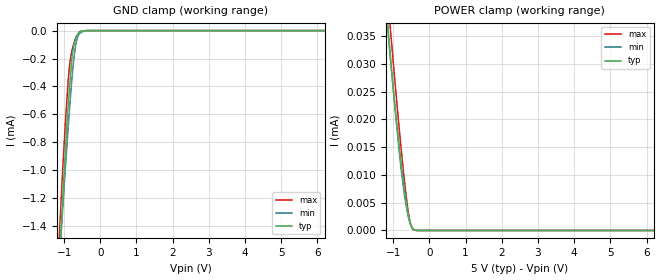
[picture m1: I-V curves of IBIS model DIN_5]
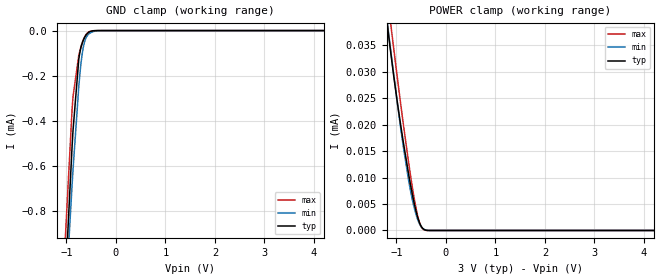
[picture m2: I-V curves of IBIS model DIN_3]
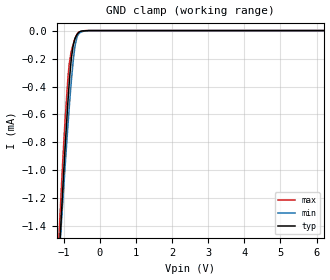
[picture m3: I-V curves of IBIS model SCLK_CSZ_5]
| Texas Instruments Incorporated
| 256 Taps, Dual Channel Digital Potentiometer with SPI Interface and Non-Volatile Memory
| Marketing part#   Voltage Range   Package-type   #pins/pkg drawing
| TPL0202-10MRTE   2.7V - 5.5V   QFN / RTE   16-pin RTE
| TPL0202-10MRUC   2.7V - 5.5V   QFN / RTE   14-pin RUC
[IBIS Ver]   4.1
[File name]   tpl0202.ibs
[File Rev]   1.0
[Date]   01/26/2012
[Source]   Model built from TISPICED simulations at:
   Texas Instruments Incorporated.
   Analog-eLab, HPA
   12500 TI Blvd
   Dallas, TX -75243
   For Support e-mail: elab_ibis@list.ti.com
[Notes]   Revision History
   Rev 1.0: 01/26/2012
   - ccomp values are based on PVT settings:
   WEAK: Low Voltage, High Temperature, Weak Process
   NOM: Nominal Voltage, Nominal Temperature, Nominal Process
   STRONG: High Voltage, Low Temperature, Fast Process
   - User may change ccomp in the order of number values as
   per end simulator used
   - C_comp although listed in numberical order of value are obtained from varying PVT conditions.
   For PVT conditions for eachspecific value, refer to the buffer description under repective [Model].
   IBIS model user is responsible for using appropriate C_comp to simulate for Signal Integrity.
   GND Clamps for DIN adn SCLK_CSZ models are non-monotonic and reflect actual circuit behavior
[Disclaimer] This model is designed as an aid for customers of Texas Instruments.
 TI and its licensors and suppliers make no warranties, either expressed
 or implied, with respect to this  model, including the warranties of
 merchantability or fitness for a particular purpose.
 The model is provided solely on an "as is" basis. The entire risk as to
 its quality and performance is with the customer.
[Copyright] (C)Copyright 2012 Texas Instruments Incorporated.
   All rights reserved.
|   Component TPL0202RTE
[Component]   TPL0202RTE
[Manufacturer]  Texas Instruments Incorporated
[Package]   |16-pin QFN RTE package
|   typ   min   max
R_pkg   0.05510   0.00044   0.09181
L_pkg   0.95615nH   0.09191nH   1.65005nH
C_pkg   0.16177pF   0.10625pF   0.22785pF
[Pin] signal_name   model_name   R_pin   L_pin   C_pin
 1   VDD   POWER   0.05907   1.02864n   0.16975p
 2   SCLK   SCLK_CSZ   0.05510   0.95615n   0.18540p
 3   DIN   DIN   0.05093   0.88345n   0.17719p
 4   CSB   SCLK_CSZ   0.05513   0.95780n   0.16776p
 5   NC   NC   0.00044   0.09191n   0.10625p
 6   NC   NC   0.00047   0.09439n   0.12678p
 7   GND   GND   0.06684   1.17207n   0.19414p
 8   NC   NC   0.00045   0.09475n   0.11241p
 9   NC   NC   0.00044   0.09191n   0.10625p
10   LB   NC   0.07541   1.33519n   0.21758p
11   WB   NC   0.08043   1.43607n   0.22785p
12   HB   NC   0.09181   1.65995n   0.21502p
13   LA   NC   0.05634   0.97306n   0.16177p
14   WA   NC   0.05052   0.87083n   0.17710p
15   HA   NC   0.05460   0.94813n   0.18216p
16   WB   NC   0.00045   0.09475n   0.11241p
|   Component TPL0202RUC
[Component]   TPL0202RUC
[Manufacturer]  Texas Instruments Incorporated
[Package]   |14-pin QFN RUC package
|   typ   min   max
R_pkg   0.03933   0.00040   0.04871
L_pkg   0.52208nH   0.16184nH   0.65360nH
C_pkg   0.12170pF   0.10389pF   0.14505pF
[Pin] signal_name   model_name   R_pin   L_pin   C_pin
 1   VDD   POWER   0.04871   0.65360n   0.11213p
 2   SCLK   SCLK_CSZ   0.03996   0.53951n   0.12170p
 3   DIN   DIN   0.04778   0.62664n   0.14505p
 4   CSB   SCLK_CSZ   0.04046   0.53776n   0.13936p
 5   GND   GND   0.04342   0.57381n   0.14139p
 6   LB   NC   0.04543   0.60528n   0.12661p
 7   WB   NC   0.03966   0.54784n   0.10459p
 8   HB   NC   0.03951   0.54862n   0.10389p
 9   NC   NC   0.00040   0.16960n   0.09156p
10   NC   NC   0.00040   0.16268n   0.10790p
11   NC   NC   0.00040   0.16184n   0.10796p
12   LA   NC   0.03864   0.52208n   0.13639p
13   WA   NC   0.03942   0.53589n   0.12085p
14   HA   NC   0.03933   0.54467n   0.10360p
[Model Selector] DIN
DIN_5 5.0V option
DIN_3 3.0V option
[Model Selector] SCLK_CSZ
SCLK_CSZ_5 5.0V option
SCLK_CSZ_3 3.0V option
| Models and submodels in the file (4): DIN_5 (Input), DIN_3 (Input), SCLK_CSZ_5 (Input), SCLK_CSZ_3 (Input)
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[Model]   DIN_5
Model_type   Input
Vinl = .8
Vinh = 2.4
|   typ   min   max
C_comp   2.500e-15   2.500e-15   2.500e-15
[Voltage Range]   5   4.5   5.5
[Temperature Range]   27   85   -40
[Power Clamp Reference]   5   4.5   5.5
[GND Clamp Reference]   -0   -0   -0
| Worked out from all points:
|   GND clamp passes 1 mA (typ) near -1.00 V on its own axis
[GND Clamp]
|   Voltage   I(typ)   I(min)   I(max)
-5V       -19.17mA   -15.47mA   -22.32mA
-1.13V    -1.634mA   -1.649mA   -1.458mA
-1.115V   -1.56mA    -1.586mA   -1.378mA
-1.055V   -1.267mA   -1.34mA    -1.071mA
-965mV    -857.7uA   -983.3uA   -655.9uA
-905mV    -591.7uA   -757.6uA   -423.1uA
-845mV    -393uA     -541.7uA   -239.4uA
-770mV    -162.2uA   -303.2uA   -129.7uA
-680mV    -55.14uA   -101.7uA   -53.32uA
-605mV    -20.37uA   -32.81uA   -17.87uA
-515mV    -3.813uA   -9.882uA   -2.785uA
9.985V    0A         0A         0A
[POWER Clamp]
|   Voltage   I(typ)   I(min)   I(max)
-5V       397.9uA    358.2uA    443.1uA
-1.25V    44.28uA    44.44uA    49.63uA
-1.13V    34.75uA    35.14uA    40.19uA
-1.085V   31.4uA     31.73uA    36.72uA
-1.025V   27.16uA    27.26uA    32.15uA
-860mV    16.74uA    15.78uA    20.07uA
-725mV    9.247uA    7.996uA    11.01uA
-635mV    4.89uA     4.194uA    5.767uA
-560mV    2.154uA    1.798uA    2.362uA
-500mV    783nA      696.5nA    719nA
-440mV    179nA      187.5nA    111.2nA
9.985V    0A         0A         0A
[Model]   DIN_3
Model_type   Input
Vinl = .8
Vinh = 2.1
|   typ   min   max
C_comp   2.500e-15   2.500e-15   2.500e-15
[Voltage Range]   3   2.7   3.3
[Temperature Range]   27   85   -40
[Power Clamp Reference]   3   2.7   3.3
[GND Clamp Reference]   -0   -0   -0
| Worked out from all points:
|   GND clamp passes 1 mA (typ) near -1.00 V on its own axis
[GND Clamp]
|   Voltage   I(typ)   I(min)   I(max)
-3V       -13.25mA   -11.89mA   -15.29mA
-1.038V   -1.185mA   -1.271mA   -988.4uA
-885mV    -512.4uA   -683uA     -348.5uA
-867mV    -444.5uA   -618.5uA   -294.2uA
-750mV    -126.9uA   -248.2uA   -109.7uA
-696mV    -66.61uA   -127.9uA   -64.3uA
-660mV    -43.25uA   -75.31uA   -41.36uA
-633mV    -30.48uA   -49.8uA    -28.17uA
-588mV    -15.58uA   -25.78uA   -13.21uA
-534mV    -5.744uA   -12.62uA   -4.363uA
-282mV    0A         -6.106nA   0A
5.991V    0A         0A         0A
[POWER Clamp]
|   Voltage   I(typ)   I(min)   I(max)
-3V       206uA      188.6uA    224.6uA
-1.2V     40.22uA    40.55uA    45.68uA
-1.146V   35.98uA    36.38uA    41.45uA
-1.065V   29.97uA    30.24uA    35.2uA
-966mV    23.23uA    23uA       27.75uA
-858mV    16.54uA    15.66uA    19.94uA
-714mV    8.596uA    7.469uA    10.33uA
-624mV    4.442uA    3.706uA    5.205uA
-561mV    2.194uA    1.834uA    2.407uA
-498mV    761.5nA    683.4nA    691.8nA
-426mV    125.3nA    140.1nA    68.79nA
5.991V    0A         0A         0A
[Model]   SCLK_CSZ_5
Model_type   Input
Vinl = .8
Vinh = 2.4
|   typ   min   max
C_comp   2.500e-15   2.500e-15   2.500e-15
[Voltage Range]   5   4.5   5.5
[Temperature Range]   27   85   -40
[Power Clamp Reference]   5   4.5   5.5
[GND Clamp Reference]   -0   -0   -0
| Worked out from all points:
|   GND clamp passes 1 mA (typ) near -1.00 V on its own axis
[GND Clamp]
|   Voltage   I(typ)   I(min)   I(max)
-5V       -19.17mA   -15.47mA   -22.32mA
-1.145V   -1.708mA   -1.711mA   -1.534mA
-1.055V   -1.265mA   -1.339mA   -1.064mA
-965mV    -845.6uA   -982.3uA   -648.1uA
-890mV    -528.4uA   -699.9uA   -357.7uA
-845mV    -362.8uA   -540.2uA   -232.9uA
-785mV    -189.7uA   -345.4uA   -140.5uA
-740mV    -108uA     -220.5uA   -100.1uA
-680mV    -51.84uA   -99.51uA   -51.34uA
-620mV    -23.35uA   -39.29uA   -21.18uA
-515mV    -3.323uA   -9.473uA   -7.07uA
9.985V    0A         0A         0A
[POWER Clamp]
|   Voltage   I(typ)   I(min)   I(max)
-5V       0A         0A         0A
0V        0A         0A         0A
10V       0A         0A         0A
